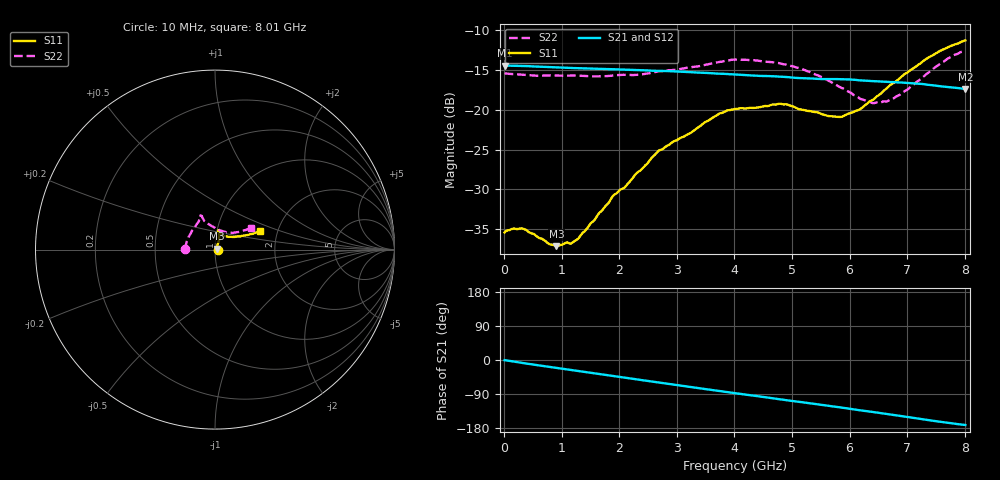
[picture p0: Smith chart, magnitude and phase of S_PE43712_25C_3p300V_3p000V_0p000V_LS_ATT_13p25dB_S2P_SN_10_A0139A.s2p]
! DEVICE ID: PE43712
! File Path: z:\PE43713\PE43713_CHAR_NOM_04292014\AMB\3p300\LS_ATT_13p25dB\PE43713_AMB_3p300V_3p000V_0p000V_LS_ATT_13p25dB_S2P_SN_10_A0139A.s2p
! Serial: 10
! Lot: A0139A
! Temp: 25C
! VDD: 3.300
! VSS: 0.000
! Control_Hi: 3.000
! Control_Lo: 0.000
! Attenuation Step: 13.25dB
! Port 1: RF1
! Port 2: RF2
! ThroughPath:1-2
! IDD: 0.000147415
! ISS: -1.744e-007
#  Hz  S  RI  R  50
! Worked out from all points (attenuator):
!   801 points, 10 MHz to 8.01 GHz, reference 50 ohm
!   highest |S21| = -14.44 dB at 20 MHz (marker M1); lowest = -17.4 dB at 8.01 GHz (marker M2)
!   lowest |S11| = -37.1 dB at 910 MHz (marker M3), VSWR 1.03, Z = 51.3 + j0.542 ohm
!   |S11| at or under -10 dB: start of sweep to end of sweep
!   |S22| runs from -19.2 to -12.6 dB; largest |S21 - S12| = 0.00069
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1e7  0.0169 0.000289  0.1896 -0.00103  0.1897 -0.000951  -0.1693 0.00111
2e7  0.0171 0.000576  0.1896 -0.00177  0.1897 -0.00176  -0.1691 0.00196
3.4e8  0.0178 0.000408  0.186 -0.0268  0.186 -0.0264  -0.1647 0.0193
9.1e8  0.0129 0.00528  0.1723 -0.0666  0.1724 -0.0666  -0.1567 0.0485
1.18e9  0.0109 0.00965  0.1631 -0.0829  0.1631 -0.083  -0.1517 0.0624
1.35e9  0.0111 0.0123  0.1568 -0.0927  0.1568 -0.0927  -0.1475 0.0697
1.9e9  0.0133 0.0258  0.1327 -0.1211  0.1327 -0.1211  -0.1312 0.099
2.11e9  0.0144 0.0297  0.1221 -0.1305  0.1222 -0.1304  -0.1258 0.1078
2.68e9  0.0225 0.0504  0.0901 -0.1504  0.0901 -0.1504  -0.1022 0.1415
3.72e9  0.023 0.0908  0.0253 -0.1667  0.0251 -0.1667  -0.0814 0.1815
4.01e9  0.0217 0.0987  0.00724 -0.1664  0.00723 -0.1664  -0.082 0.1896
4.79e9  0.0197 0.1074  -0.038 -0.1568  -0.0381 -0.157  -0.0725 0.1818
5.35e9  0.0302 0.0925  -0.0664 -0.1424  -0.0664 -0.1423  -0.0594 0.1598
5.64e9  0.0405 0.0817  -0.0795 -0.1341  -0.0795 -0.1341  -0.0418 0.1459
5.88e9  0.0512 0.075  -0.0913 -0.1258  -0.0911 -0.1258  -0.0232 0.1343
6.17e9  0.0702 0.0716  -0.1033 -0.1129  -0.1031 -0.1131  0.00438 0.1179
6.38e9  0.0889 0.0719  -0.1102 -0.1038  -0.11 -0.1038  0.027 0.1075
6.68e9  0.1202 0.0721  -0.1196 -0.0896  -0.1194 -0.0896  0.0622 0.096
7e9  0.153 0.0769  -0.1281 -0.0732  -0.1279 -0.0732  0.0958 0.0931
7.37e9  0.1948 0.0856  -0.1336 -0.0522  -0.1334 -0.0522  0.1386 0.1004
7.72e9  0.2296 0.095  -0.1346 -0.0336  -0.1346 -0.0337  0.1785 0.1128
8.01e9  0.2509 0.1062  -0.1336 -0.0197  -0.1334 -0.02  0.1994 0.1212
